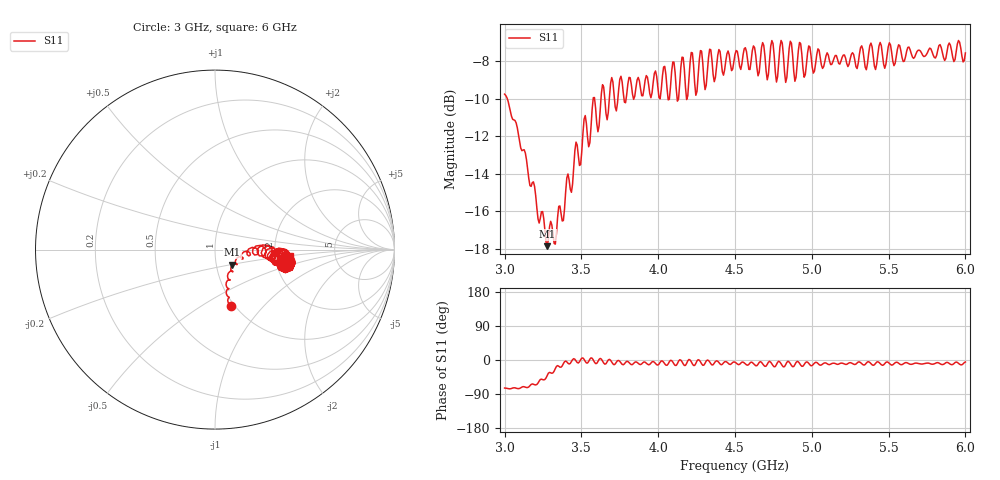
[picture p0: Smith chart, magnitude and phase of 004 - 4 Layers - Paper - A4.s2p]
!  02/07/2025  15:41:41
! Ref Plane: 0.000 mm
# MHZ S MA R  50
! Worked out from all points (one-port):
!   401 points, 3 GHz to 6 GHz, reference 50 ohm
!   lowest |S11| = -17.9 dB at 3.277 GHz (marker M1), VSWR 1.29, Z = 59.8 - j10.1 ohm
!   |S11| at or under -10 dB: 3.017 GHz to 3.577 GHz (559.5 MHz wide, 17 % of centre); 3.586 GHz to 3.628 GHz (41.77 MHz wide, 1.16 % of centre); 3.652 GHz to 3.682 GHz (29.39 MHz wide, 0.801 % of centre)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
3000  0.3252 -74.0
3277.5  0.128 -40.6
3375  0.1494 -15.6
3525  0.2852 -3.6
3750  0.3563 -3.7
4065  0.314 -10.3
4095  0.396 -5.3
4125  0.3115 -9.6
4155  0.4079 -4.7
4185  0.3146 -9.0
4215  0.4199 -4.5
4245  0.3229 -9.1
4275  0.4248 -4.7
4305  0.3344 -8.6
4335  0.4284 -5.0
4500  0.4149 -5.8
4695  0.4105 -16.8
4725  0.4017 -3.7
4755  0.4121 -18.0
4785  0.3981 -3.5
4815  0.4131 -18.1
4845  0.3944 -3.6
4875  0.4133 -17.7
4905  0.3913 -3.8
4935  0.4158 -16.7
5250  0.4037 -7.0
5625  0.4331 -8.2
6000  0.4186 -5.2
